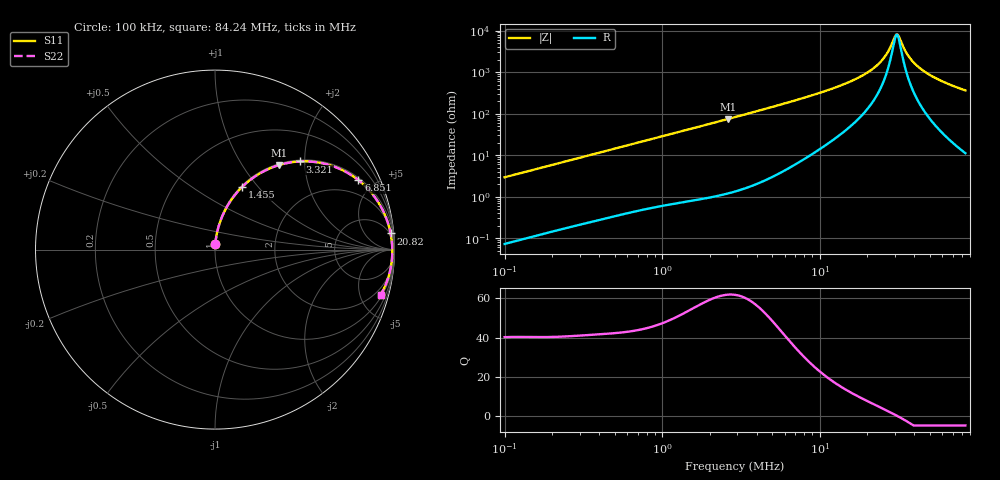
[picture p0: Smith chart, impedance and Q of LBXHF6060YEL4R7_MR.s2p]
! LBXHF6060YEL4R7_MR  S-PARAMETER MODEL  ( General Type )
! Model Generated by TAIYO YUDEN Corporation (http://www.ty-top.com)
! Version 1.0
! TAIYO YUDEN Control No. 200120NI43SB-FBB
! Copyright(c) 2020 TAIYO YUDEN CO.,LTD. All Rights Reserved.
! Product Description (link to TY-COMPAS)
! https://ds.yuden.co.jp/TYCOMPAS/or/detail?pn=LBXHF6060YEL4R7MMR&u=M
! Products Name : Inductors
! Characteristics :
!  Inductance : 4.7 uH , SRF(min) : 22 MHz , DC Resistance(max) : 0.036 Ohm
!  Rated Current : Saturation :6000 mA , Temp Rise : 2200 mA
!  Case Size : 6.0 x 6.0 / 0.236 x 0.236 [mm/inch] , Thickness : 4.5 / 0.177 [mm/inch]
!  (Conditions: Temperature = 25 degC , DC Bias Current/Voltage = 0A / 0V)
! External Node Assignments :
!  1  o---GGG---o  2
! GND o---------o GND
! Frequency Range : 0.1MHz  -  84.23641MHz  [ 402 STEP ]
# MHz S RI R 50
! Freq[MHz].  S11 Real  S11 Imag  S21 Real  S21 Imag  S12 Real  S12 Imag  S22 Real  S22 Imag
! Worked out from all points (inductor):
!   401 points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, 100 kHz to 84.24 MHz, reference 50 ohm
!   read as one part in series: L = 4.66 uH near 103.4 kHz
!   highest Q = 62 at 2.623 MHz (marker M1), where L = 4.51 uH
!   self-resonance near 30.67 MHz
!   S11 on the Smith chart (normalised r, x): 100 kHz: 1.00, +0.06; 1.455 MHz: 1.02, +0.82; 3.321 MHz: 1.03, +1.89; 6.851 MHz: 1.11, +4.07; 20.82 MHz: 4, +21; 84.24 MHz: 1.22, -7.23
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0.1  0.00159 0.0293  0.9984 -0.0293  0.9984 -0.0293  0.00159 0.0293
0.309045  0.01 0.0882  0.99 -0.0882  0.99 -0.0882  0.01 0.0882
0.955086  0.0732 0.25  0.9268 -0.25  0.9268 -0.25  0.0732 0.25
1.455078  0.1496 0.3474  0.8504 -0.3474  0.8504 -0.3474  0.1496 0.3474
2.623418  0.3584 0.4715  0.6416 -0.4715  0.6416 -0.4715  0.3584 0.4715
2.902351  0.4061 0.4831  0.5939 -0.4831  0.5939 -0.4831  0.4061 0.4831
3.320932  0.4727 0.4911  0.5273 -0.4911  0.5273 -0.4911  0.4727 0.4911
4.650878  0.6401 0.4703  0.3599 -0.4703  0.3599 -0.4703  0.6401 0.4703
6.850956  0.7987 0.3872  0.2013 -0.3872  0.2013 -0.3872  0.7987 0.3872
8.96956  0.8753 0.3118  0.1247 -0.3118  0.1247 -0.3118  0.8753 0.3118
14.86564  0.9551 0.1724  0.0449 -0.1724  0.0449 -0.1724  0.9551 0.1724
20.81894  0.9784 0.0899  0.0216 -0.0899  0.0216 -0.0899  0.9784 0.0899
24.63747  0.9844 0.0512  0.0156 -0.0512  0.0156 -0.0512  0.9844 0.0512
27.71995  0.9868 0.0246  0.0132 -0.0246  0.0132 -0.0246  0.9868 0.0246
30.15512  0.9877 0.00567  0.0123 -0.00567  0.0123 -0.00567  0.9877 0.00567
31.18808  0.9879 -0.00192  0.0121 0.00192  0.0121 0.00192  0.9879 -0.00192
32.25642  0.9879 -0.00951  0.0121 0.00951  0.0121 0.00951  0.9879 -0.00951
34.50413  0.9876 -0.0248  0.0124 0.0248  0.0124 0.0248  0.9876 -0.0248
36.90848  0.9869 -0.0402  0.0131 0.0402  0.0131 0.0402  0.9869 -0.0402
43.67809  0.9828 -0.0795  0.0172 0.0795  0.0172 0.0795  0.9828 -0.0795
57.1852  0.9682 -0.1464  0.0318 0.1464  0.0318 0.1464  0.9682 -0.1464
84.23641  0.9222 -0.2528  0.0778 0.2528  0.0778 0.2528  0.9222 -0.2528
